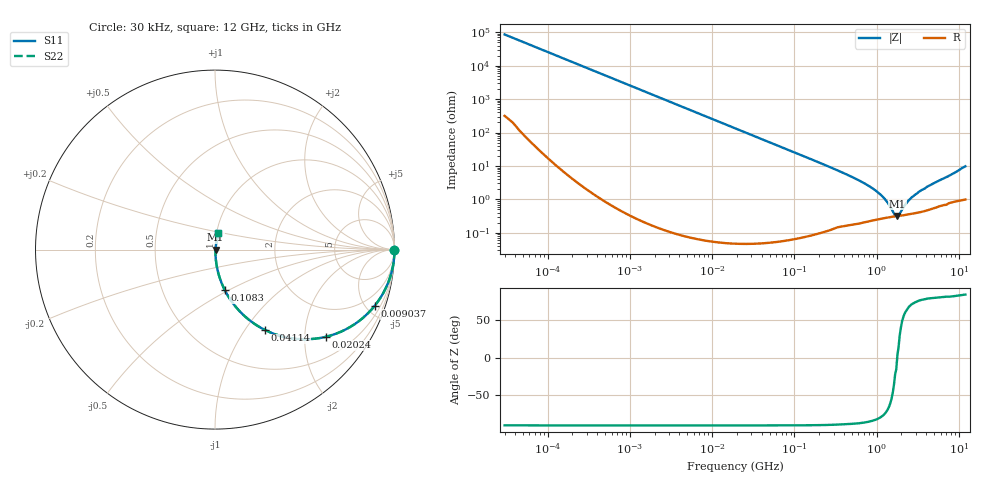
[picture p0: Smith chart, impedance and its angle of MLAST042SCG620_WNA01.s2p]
! MLAST042SCG620_WNA01  S-PARAMETER MODEL  ( General Type )
! Model Generated by TAIYO YUDEN Corporation (http://www.ty-top.com)
! Version 1.0
! TAIYO YUDEN Control No. 150820
! Copyright(c) 2015 TAIYO YUDEN CO.,LTD. All Rights Reserved.
! Product Description (link to TY-COMPAS)
! https://ds.yuden.co.jp/TYCOMPAS/or/detail?pn=MLAST042SCG620JWNA01&u=M
! Products Name : Multilayer Ceramic Capacitors
! Characteristics :
!  Capacitance : 62 pF , Rated Voltage : 25V , TCC : CG / C0G
!  Case Size : 0.4 x 0.2 / 0.016 x 0.008 [mm/inch] , Thickness : 0.2 / 0.008 [mm/inch]
!  (Conditions: Temperature = 25 degC , DC Bias Current/Voltage = 0A / 0V)
! External Node Assignments :
!  1  o---| |---o  2
! GND o---------o GND
! Frequency Range : 0.03MHz  -  12000MHz  [ 401 STEP ]
# MHz S RI R 50
! Freq[MHz].  S11 Real  S11 Imag  S21 Real  S21 Imag  S12 Real  S12 Imag  S22 Real  S22 Imag
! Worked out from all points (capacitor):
!   401 points, 30 kHz to 12 GHz, reference 50 ohm
!   read as one part in series: C = 62 pF near 32 kHz
!   lowest |Z| = 320 mohm at 1.79 GHz (marker M1)
!   series resonance near 1.779 GHz, so ESL is about 130 pH
!   S11 on the Smith chart (normalised r, x): 30 kHz: open; 9.037 MHz: 1.00, -5.68; 20.24 MHz: 1.00, -2.54; 41.14 MHz: 1.00, -1.25; 108.3 MHz: 1.00, -0.47; 12 GHz: 1.02, +0.19
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0.03  1 -0.00117  5.68e-06 0.00117  5.68e-06 0.00117  1 -0.00117
0.260295  0.9999 -0.0101  0.000105 0.0101  0.000105 0.0101  0.9999 -0.0101
2.258455  0.9923 -0.0873  0.00769 0.0873  0.00769 0.0873  0.9923 -0.0873
5.057549  0.9626 -0.1896  0.0374 0.1896  0.0374 0.1896  0.9626 -0.1896
9.037177  0.8897 -0.3132  0.1103 0.3132  0.1103 0.3132  0.8897 -0.3132
18.97367  0.6466 -0.4779  0.3534 0.4779  0.3534 0.4779  0.6466 -0.4779
20.23772  0.6166 -0.486  0.3834 0.486  0.3834 0.486  0.6166 -0.486
28.85481  0.4417 -0.4963  0.5583 0.4963  0.5583 0.4963  0.4417 -0.4963
41.141  0.2802 -0.4487  0.7198 0.4487  0.7198 0.4487  0.2802 -0.4487
64.61702  0.1363 -0.3425  0.8637 0.3425  0.8637 0.3425  0.1363 -0.3425
108.2504  0.0534 -0.2235  0.9466 0.2235  0.9466 0.2235  0.0534 -0.2235
164.6252  0.0241 -0.1507  0.9759 0.1507  0.9759 0.1507  0.0241 -0.1507
419.4166  0.00493 -0.0573  0.9951 0.0573  0.9951 0.0573  0.00493 -0.0573
749.4426  0.0029 -0.0278  0.9971 0.0278  0.9971 0.0278  0.0029 -0.0278
1103.571  0.00279 -0.014  0.9972 0.014  0.9972 0.014  0.00279 -0.014
1428.372  0.00296 -0.00599  0.997 0.00599  0.997 0.00599  0.00296 -0.00599
1625.032  0.00308 -0.0022  0.9969 0.0022  0.9969 0.0022  0.00308 -0.0022
1790.1  0.00318 0.000211  0.9968 -0.000211  0.9968 -0.000211  0.00318 0.000211
1909.359  0.00324 0.00187  0.9968 -0.00187  0.9968 -0.00187  0.00324 0.00187
2471.32  0.00365 0.00877  0.9964 -0.00877  0.9964 -0.00877  0.00365 0.00877
3198.675  0.00425 0.0156  0.9958 -0.0156  0.9958 -0.0156  0.00425 0.0156
12000  0.0189 0.0946  0.9811 -0.0946  0.9811 -0.0946  0.0189 0.0946
